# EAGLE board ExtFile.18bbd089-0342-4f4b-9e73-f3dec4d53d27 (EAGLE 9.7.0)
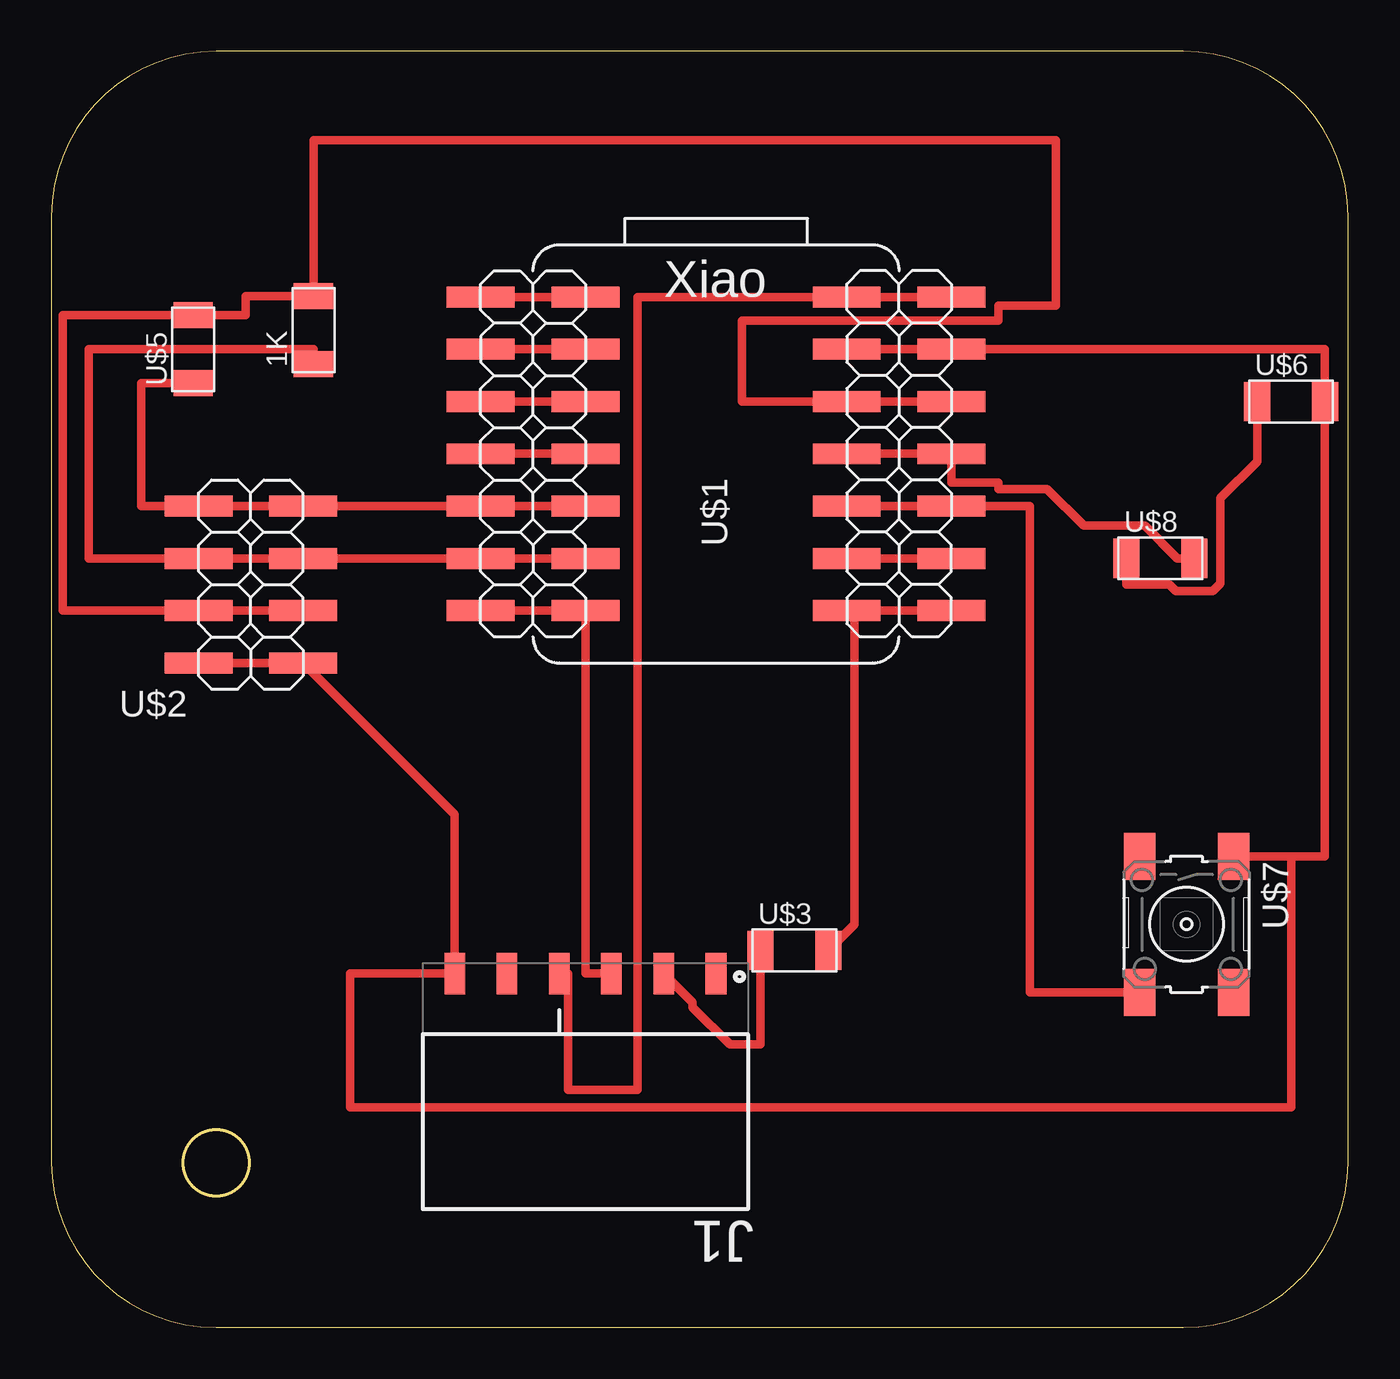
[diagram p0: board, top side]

Size 63 x 62 mm. Coordinates in mm from the lower left corner, seen from the top.
Outline: 8,62 arc90 0,54 0,8 arc90 8,0 55,0 arc90 63,8 63,54 arc90 55,62 8,62
Outline: circle at 8,8 radius 1.6
Copper layers (1*16): Top / Bottom
Stack-up Default Layer Stack: Top User Defined 0.035mm / Dielectric-1 User Defined 1.5mm / Bottom User Defined 0.035mm
Design rules: minimum drill size all 0.8mm, minimum drill size 0.35mm, minimum copper width all 16mil, minimum copper width 6mil, keepout clearance 0mil, drill distance 6mil, via restrict clearance 0mil, dimension clearance 40mil, restrict clearance 0mil, copper clearance all to all 17mil, copper clearance wire_polygon to wire_polygon 6mil, copper clearance wire_polygon to pad_smd 6mil, copper clearance wire_polygon to via 6mil, copper clearance pad_smd to pad_smd 6mil, copper clearance pad_smd to via 6mil, copper clearance via to via 6mil, copper clearance smd to pad (same net) 6mil, copper clearance smd to via (same net) 6mil, copper clearance smd to smd (same net) 6mil

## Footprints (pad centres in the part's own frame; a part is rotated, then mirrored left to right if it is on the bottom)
R1206FAB = smd 1.27 x 1.905: 1 -1.651,0; 2 1.651,0
1X6_RIGHTANGLE_PINSOCKET = smd 1 x 2: 1 -6.35,-5.225; 2 -3.81,-5.225; 3 -1.27,-5.225; 4 1.27,-5.225; 5 3.81,-5.225; 6 6.35,-5.225
2X07X2_SMD = smd 3.302 x 1.016: 1 -11.43,7.62; 3 -11.43,5.08; 5 -11.43,2.54; 7 -11.43,0; 9 -11.43,-2.54; 11 -11.43,-5.08; 13 -11.43,-7.62; 16 11.43,7.62; 18 11.43,5.08; 20 11.43,2.54; 22 11.43,0; 24 11.43,-2.54; 26 11.43,-5.08; 28 11.43,-7.62; +3V3 6.35,2.54; +5V 6.35,7.62; GND 6.35,5.08; P0 -6.35,-7.62; P1 6.35,-7.62; P2 6.35,-5.08; P3 6.35,0; P4 6.35,-2.54; P6 -6.35,-2.54; P7 -6.35,-5.08; P26 -6.35,7.62; P27 -6.35,5.08; P28 -6.35,2.54; P29 -6.35,0
2X04SMD = smd 1.016 x 3.302: 1 -1.27,-3.81; 2 -1.27,1.27; 3 1.27,-3.81; 4 1.27,1.27; 5 3.81,-3.81; 6 3.81,1.27; 7 6.35,-3.81; 8 6.35,1.27
LED1206FAB = smd 1.27 x 1.905: 1 -1.651,0; 2 1.651,0
6MM_SWITCH = smd 2.286 x 1.524: 1 -3.302,2.286; 2 3.302,2.286; 3 -3.302,-2.286; 4 3.302,-2.286

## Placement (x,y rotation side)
1K  RES_FAB  [R1206FAB]  12.73,48.46 90 top
J1  1X6_RIGHTANGLE_PINSOCKET  [1X6_RIGHTANGLE_PINSOCKET]  25.94,11.97 180 top
U$1  XIAO_RP2040_2X7X2_SMD  [2X07X2_SMD]  32.29,42.45 0 top
U$2  PINHEADER2X04_SMD  [2X04SMD]  8.41,33.56 90 top
U$3  1K  [R1206FAB]  36.1,18.32 0 top
U$5  1K  [R1206FAB]  6.89,47.53 90 top
U$6  LED_FAB  [LED1206FAB]  60.23,44.99 0 top
U$7  SWITCH_TACT  [6MM_SWITCH]  55.15,19.59 270 top
U$8  1K  [R1206FAB]  53.88,37.37 0 top

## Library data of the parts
1K U$3 U$5 U$8 = RES_FAB
J1 = 1x6_RightAngle_PinSocket; MANUFACTURER: GCT
U$1 = xiao_RP2040_2x07x2P
U$2 = PinHeader_Socket_2x04_SMD
U$6 = LED_FAB
U$7 = SWITCH_TACT

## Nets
+3V3: 1K.2 U$1.20 U$1.+3V3 U$2.3 U$2.4 U$5.2
+5V: J1.4 U$1.16 U$1.+5V
A0_D0: U$1.1 U$1.P26
A1_D1: U$1.3 U$1.P27
A2_D2: U$1.5 U$1.P28
A3_D3: U$1.7 U$1.P29
BTN_PIN: U$1.24 U$1.P4 U$7.4
DB: U$1.26 U$1.P2
GND: J1.6 U$1.18 U$1.GND U$2.1 U$2.2 U$6.2 U$7.1
LED_PIN: U$1.22 U$1.P3 U$8.2
N$1: J1.2 U$3.1
N$3: U$6.1 U$8.1
RX_PIN: U$1.28 U$1.P1 U$3.2
SCL: 1K.1 U$1.11 U$1.P7 U$2.5 U$2.6
SDA: U$1.9 U$1.P6 U$2.7 U$2.8 U$5.1
TX_PIN: J1.3 U$1.13 U$1.P0

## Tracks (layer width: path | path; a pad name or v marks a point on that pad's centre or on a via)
+3V3
  Top 0.406: U$2.3 U$2.4 0.54,34.83 0.54,49.18 U$5.2 9.43,49.18 9.43,50.11 1K.2 12.73,57.69 48.8,57.69 48.8,49.64 46.01,49.64 46.01,48.93 33.56,48.93 33.56,44.99 U$1.+3V3 U$1.20
+5V
  Top 0.406: J1.4 25.1,17.2 25.1,11.54 28.48,11.54 28.48,50.07 U$1.+5V U$1.16
A0_D0
  Top 0.406: U$1.P26 U$1.1
A1_D1
  Top 0.406: U$1.P27 U$1.3
A2_D2
  Top 0.406: U$1.P28 U$1.5
A3_D3
  Top 0.406: U$1.P29 U$1.7
BTN_PIN
  Top 0.406: U$7.4 47.53,16.29 47.53,39.91 U$1.24 U$1.P4
DB
  Top 0.406: U$1.26 U$1.P2
GND
  Top 0.406: U$2.2 U$2.1 19.59,24.92 J1.6 14.51,17.2 14.51,10.7 60.23,10.7 60.23,22.89 U$7.1 61.88,22.89 U$6.2 61.88,47.53 U$1.18 U$1.GND
LED_PIN
  Top 0.406: U$8.2 54.72,37.37 53.13,38.96 50.16,38.96 48.37,40.75 46.01,40.75 46.01,41.05 43.72,41.05 U$1.22 U$1.P3
N$1
  Top 0.406: U$3.1 34.45,13.75 32.97,13.75 31.16,15.56 31.16,15.79 J1.2
N$3
  Top 0.406: U$6.1 58.58,42.07 56.8,40.29 56.8,36.15 56.43,35.78 54.63,35.78 54.31,36.1 52.23,36.1 U$8.1
RX_PIN
  Top 0.406: U$3.2 39.02,19.59 39.02,34.45 U$1.P1 U$1.28
SCL
  Top 0.406: 1K.1 12.73,47.53 1.81,47.53 1.81,37.37 U$2.6 U$2.5 U$1.11 U$1.P7
SDA
  Top 0.406: U$1.P6 U$1.9 U$2.7 U$2.8 4.35,39.91 4.35,45.88 U$5.1
TX_PIN
  Top 0.406: J1.3 25.94,17.2 U$1.P0 U$1.13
